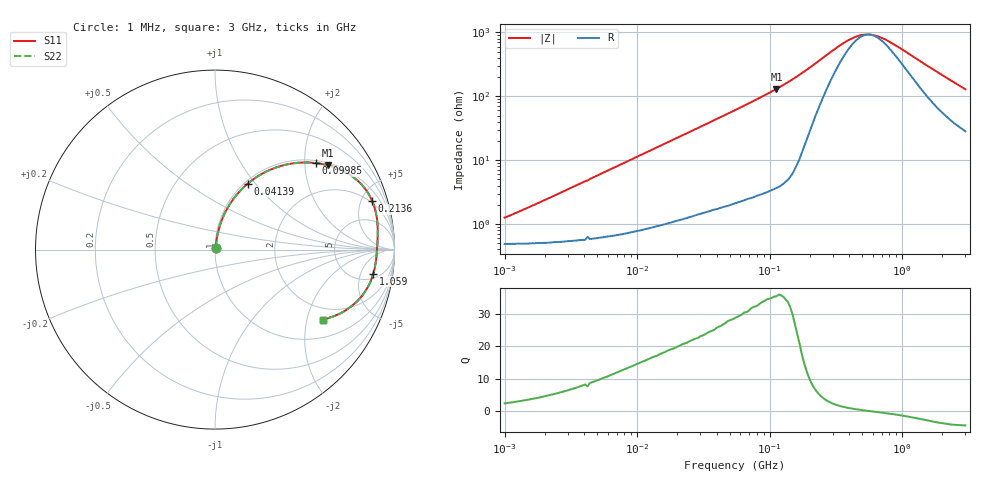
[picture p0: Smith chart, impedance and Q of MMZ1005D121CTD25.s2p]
! S-Parameter Data Generated by TDK Corporation
! Copyright(C) 2025 TDK Corporation.
! All Rights Reserved.
! TDK P/N: MMZ1005D121CTD25 (Chip Bead)
! Property: |Z|=120ohm at 100MHz
! Size(LxWxT): 1x0.5x0.5mm
! Model Type: s2p (Touchstone File Format Version 1.0)
! Frequency: DC=Yes Start=1MHz Stop=3000MHz 202points Log-sweep
! Model Generated on Feb. 6, 2025
! Terms and conditions regarding TDK Simulation Models:
! 1)This simulation model is being provided solely for informational
!  purposes. Please refer to the specifications of the products in
!  terms of detailed characteristics of such products.
! 2)In no event shall TDK Corporation of any of its subsidiaries be
!  liable for any loss or damage arising, directly or indirectly,
!  from any information contained in this simulation model, including,
!  but not limited to loss or damages arising from any inaccuracies,
!  omissions or errors in connection with such information.
! 3)Any and all copyrights on this simulation model are owned by
!  TDK Corporation.  Duplication or redistribution of this simulation
!  model without prior written permission from TDK Corporation
!  is prohibited.
! 4)This simulation model is subject to any modification or change
!  without any prior notice.
! 5)Neither TDK Corporation nor any of its subsidiaries shall make any
!  warranty, express or implied, including but not limited to the
!  correctness, implied warranties of merchantability and fitness for
!  a particular purpose with respect to this simulation models.
! 6)The use of this simulation model shall be deemed to have consented
!  to the terms and conditions hereof.
! Port Assignments:
!  1 ---@@@--- 2
! Applicable Conditions:
!  Temperature = 25 degC
!  DC Bias Current = 0 A
!  Small Signal Operation
# Hz S MA R 50
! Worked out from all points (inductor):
!   201 points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, 1 MHz to 3 GHz, reference 50 ohm
!   read as one part in series: L = 184 nH near 1.323 MHz
!   highest Q = 35.4 at 112.6 MHz (marker M1), where L = 185 nH
!   self-resonance near 565.2 MHz
!   S11 on the Smith chart (normalised r, x): 1 MHz: 1.01, +0.02; 41.39 MHz: 1.04, +0.91; 99.85 MHz: 1.07, +2.28; 213.6 MHz: 1.81, +6.12; 1.059 GHz: 6, -8; 3 GHz: 1.57, -2.51
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1000000  0.01254 66.6  0.9951 -0.7  0.9951 -0.7  0.01254 66.6
3900413  0.04476 80.3  0.9934 -2.5  0.9934 -2.5  0.04476 80.3
8017732  0.09007 80.4  0.989 -5.2  0.989 -5.2  0.09007 80.4
1.461624e7  0.1604 77.5  0.9779 -9.2  0.9779 -9.2  0.1604 77.5
2.559965e7  0.2701 71.7  0.9505 -15.7  0.9505 -15.7  0.2701 71.7
4.138676e7  0.4101 63.6  0.8965 -24.2  0.8965 -24.2  0.4101 63.6
5.477226e7  0.5106 57.3  0.8422 -30.7  0.8422 -30.7  0.5106 57.3
7.544761e7  0.6351 48.8  0.753 -39.4  0.753 -39.4  0.6351 48.8
9.984923e7  0.7413 40.5  0.6502 -47.8  0.6502 -47.8  0.7413 40.5
1.125904e8  0.7834 36.8  0.5999 -51.5  0.5999 -51.5  0.7834 36.8
1.614254e8  0.8846 25.5  0.4306 -62.1  0.4306 -62.1  0.8846 25.5
2.136344e8  0.9166 17.1  0.297 -65.3  0.297 -65.3  0.9166 17.1
3.594878e8  0.9124 6.1  0.1347 -46.4  0.1347 -46.4  0.9124 6.1
4.75755e8  0.9054 2.2  0.1012 -19.7  0.1012 -19.7  0.9054 2.2
5.364635e8  0.9034 0.7  0.09727 -6.2  0.09727 -6.2  0.9034 0.7
6.049187e8  0.9016 -0.8  0.09933 7.5  0.09933 7.5  0.9016 -0.8
8.005644e8  0.8982 -4.5  0.1257 33.8  0.1257 33.8  0.8982 -4.5
1.059487e9  0.8922 -8.6  0.1782 48.6  0.1782 48.6  0.8922 -8.6
1.402151e9  0.8768 -13.7  0.2557 54.6  0.2557 54.6  0.8768 -13.7
1.782824e9  0.8492 -19.0  0.3398 54.5  0.3398 54.5  0.8492 -19.0
2.266846e9  0.8019 -25.0  0.4359 51.1  0.4359 51.1  0.8019 -25.0
3e9  0.7169 -32.9  0.5572 44.4  0.5572 44.4  0.7169 -32.9
